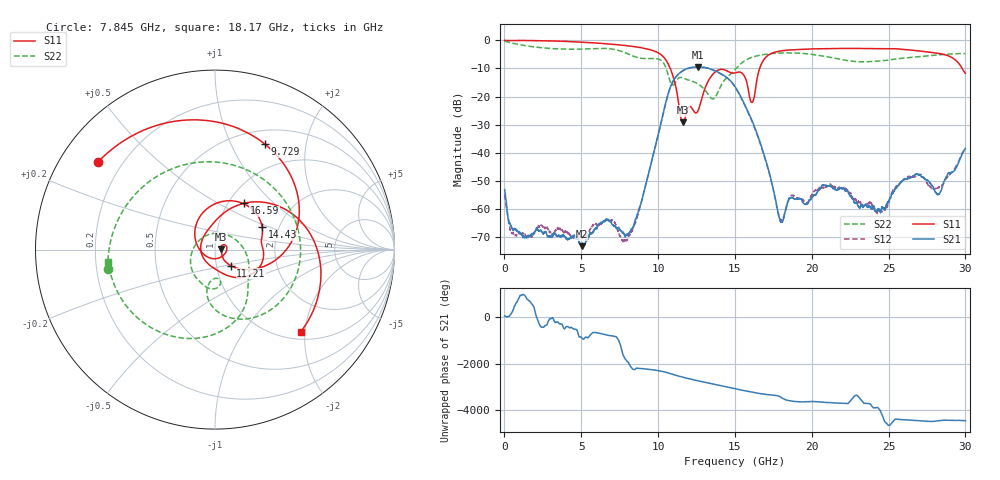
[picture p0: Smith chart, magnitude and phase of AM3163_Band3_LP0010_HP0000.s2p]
!Agilent Technologies,E8364B,MY43040894,A.07.50.67
!Agilent E8364B: A.07.50.67
!Date: Thursday, August 20, 2020 12:13:41
!Correction: S11(Full 2 Port(1,2))
!S21(Full 2 Port(1,2))
!S12(Full 2 Port(1,2))
!S22(Full 2 Port(1,2))
!S2P File: Measurements: S11, S21, S12, S22:
# Hz S  dB  R 50
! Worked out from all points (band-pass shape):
!   3201 points, 10 MHz to 30 GHz, reference 50 ohm
!   highest |S21| = -9.42 dB at 12.62 GHz (marker M1); lowest = -73.4 dB at 5.015 GHz (marker M2)
!   |S21| within 3 dB of the highest: 11.24 GHz to 14.26 GHz (3.024 GHz wide, 23.7 % of centre)
!   lowest |S11| = -29.2 dB at 11.63 GHz (marker M3), VSWR 1.07, Z = 53.6 + j0.349 ohm
!   |S11| at or under -10 dB: 10.79 GHz to 16.61 GHz (5.814 GHz wide, 42.4 % of centre); 29.79 GHz to end of sweep
!   |S22| runs from -20.9 to -0.3 dB; largest |S21 - S12| = 0.0042
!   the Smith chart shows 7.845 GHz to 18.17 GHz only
!   S11 on the Smith chart (normalised r, x): 7.845 GHz: 0.11, +0.33; 9.729 GHz: 0.66, +1.35; 11.21 GHz: 1.17, -0.21; 14.43 GHz: 1.64, +0.44; 16.59 GHz: 1.18, +0.67; 18.17 GHz: 1.17, -1.90
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1e7  0.01 -1.9  -53.21 54.9  -54.96 146.8  -0.29 -6.9
9.753031e8  -0.01 -26.7  -68.79 142.5  -68.62 -121.4  -1.48 -85.5
2.25925e9  -0.07 -62.0  -68.10 67.9  -66.60 -27.1  -2.50 -169.5
5.014581e9  -0.61 -135.7  -73.41 -145.7  -70.10 25.4  -3.08 43.5
6.795238e9  -1.24 175.4  -64.07 -63.6  -64.25 84.7  -2.92 -75.1
7.844888e9  -1.78 143.1  -69.82 32.7  -70.84 -151.3  -4.34 -169.8
8.735216e9  -2.42 111.2  -60.27 -34.3  -61.28 -36.4  -6.17 95.1
9.728634e9  -3.74 64.8  -39.96 -104.7  -40.04 -105.2  -6.43 -9.2
1.000979e10  -4.43 47.6  -33.55 -133.0  -33.69 -133.6  -6.63 -38.1
1.120939e10  -18.06 -45.7  -12.61 17.4  -12.68 17.4  -14.17 -81.4
1.163112e10  -29.19 5.4  -10.70 -58.1  -10.80 -58.1  -13.38 -103.2
1.261517e10  -24.85 -131.8  -9.42 149.0  -9.47 149.3  -15.59 -142.5
1.443332e10  -10.73 25.3  -13.05 -101.9  -13.18 -101.9  -13.43 -27.3
1.5005e10  -11.57 3.7  -16.46 174.1  -16.62 174.3  -10.44 -52.5
1.611088e10  -22.11 -168.0  -28.61 26.0  -28.87 26.5  -6.01 -100.2
1.658885e10  -10.29 57.7  -35.55 -30.8  -35.93 -29.1  -5.30 -118.8
1.817269e10  -3.58 -43.8  -63.20 98.6  -62.66 104.6  -4.44 -173.4
2.000958e10  -3.02 -100.2  -56.05 -15.9  -54.91 -25.7  -4.95 122.2
2.249313e10  -2.82 -157.6  -55.58 -8.0  -54.26 -127.2  -7.31 11.7
2.500479e10  -3.00 144.2  -57.72 43.3  -57.32 -46.0  -6.98 -103.0
2.827558e10  -4.63 50.1  -54.68 -114.9  -52.29 -112.8  -5.14 148.2
3e10  -11.74 -29.4  -38.54 -118.5  -38.40 -114.3  -4.66 99.3
